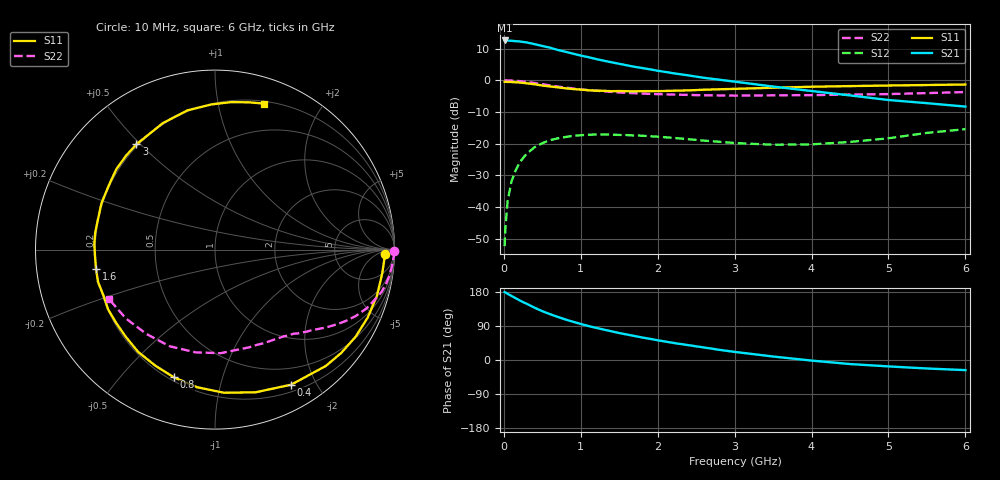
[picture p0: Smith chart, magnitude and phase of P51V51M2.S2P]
! SIEMENS Small Signal Semiconductors
! BFP183
! Si NPN RF Bipolar Junction Transistor in SOT143
! VCE = 1.5 V  IC = 1.2 mA
! Common Emitter S-Parameters:  March  1996
# GHz  S  MA  R  50
!  f  S11  S21  S12  S22
! GHz  MAG  ANG  MAG  ANG  MAG  ANG  MAG  ANG
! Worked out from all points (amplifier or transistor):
!   36 points, 10 MHz to 6 GHz, reference 50 ohm
!   highest |S21| = 12.6 dB at 10 MHz (marker M1)
!   |S21| within 3 dB of that: start of sweep to 700 MHz
!   unconditionally stable (mu >= 1): 2.338 GHz to end of sweep
!   at 250 MHz: K = 0.10, MSG = 18.3 dB, |S12| = -24.5 dB
!   at 1.4 GHz: K = 0.58, MSG = 11.4 dB, |S12| = -17.2 dB
!   at 6 GHz: K = 1.08, MAG = 1.9 dB, |S12| = -15.4 dB
!   S11 on the Smith chart (normalised r, x): 10 MHz: 31, -14; 400 MHz: 0.28, -1.68; 800 MHz: 0.22, -0.71; 1.6 GHz: 0.20, -0.08; 3 GHz: 0.19, +0.49; 6 GHz: 0.22, +1.37
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0.01  0.9475 -1.4  4.256 179.2  0.0024 85.7  1 -0.6
0.02  0.9448 -3.4  4.248 178.4  0.0046 83.8  0.9988 -1.2
0.05  0.9412 -8.0  4.245 174.5  0.0126 86.7  0.995 -2.9
0.1  0.9384 -15.9  4.206 169.1  0.0252 80.2  0.9888 -5.8
0.2  0.9219 -31.7  4.118 158.0  0.0492 71.5  0.9712 -11.5
0.25  0.909 -39.3  4.031 152.7  0.0593 66.9  0.9573 -14.3
0.3  0.8953 -46.4  3.952 148.1  0.0698 62.7  0.9385 -16.7
0.4  0.864 -60.6  3.72 137.9  0.0878 54.9  0.9058 -21.2
0.5  0.8266 -74.1  3.482 128.8  0.1017 47.4  0.8677 -25.2
0.6  0.7992 -86.4  3.277 121.0  0.1131 41.0  0.8303 -28.6
0.8  0.7475 -107.8  2.824 107.0  0.1271 30.4  0.7671 -34.0
0.9  0.7273 -117.2  2.631 100.9  0.1328 26.1  0.7426 -36.1
1.1  0.6951 -135.6  2.317 89.6  0.138 18.6  0.699 -40.1
1.3  0.6823 -150.8  2.038 80.1  0.1391 12.2  0.6685 -43.7
1.6  0.6716 -170.7  1.722 67.2  0.1362 5.2  0.634 -48.3
1.8  0.6731 177.5  1.561 59.3  0.1332 2.0  0.6162 -51.6
2.2  0.6836 157.6  1.293 45.2  0.1232 -3.0  0.5949 -58.8
3  0.732 126.7  0.952 21.4  0.1022 -3.0  0.5725 -75.3
3.5  0.7626 112.3  0.796 9.2  0.096 2.9  0.578 -86.9
4.5  0.8092 91.3  0.577 -10.7  0.1062 17.8  0.5949 -115.2
5.5  0.8416 77.2  0.435 -22.4  0.1476 22.8  0.6276 -142.3
6  0.8577 71.5  0.384 -26.7  0.1691 20.1  0.6519 -155.0
